(* Logix 5000 AddOnInstructionDefinition export AMCI_3204_AOP_Reset_Errors; software revision 20.03 *)

ADD_ON_INSTRUCTION AMCI_3204_AOP_Reset_Errors   (* revision 1.0, vendor AMCI, ExecuteEnableInFalse *)
VAR_INPUT
   axis_status_bits : INT; {required}
   channel_number : INT; {required}
END_VAR
VAR_IN_OUT
   AMCI_3204_output_data : AM:1756_3204:O:0; {required}
END_VAR
VAR_OUTPUT
   EN : BOOL; {access Read Only, visible}
END_VAR
VAR
   command_data_block : DINT[8]; {access None}
END_VAR

ROUTINE EnableInFalse   (* ladder *)
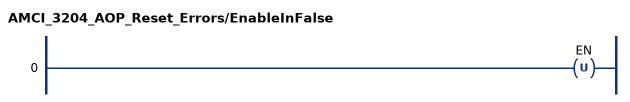
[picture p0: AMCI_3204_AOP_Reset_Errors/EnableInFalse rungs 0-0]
   0: OTU(EN);
END_ROUTINE

ROUTINE Logic   (* ladder *)
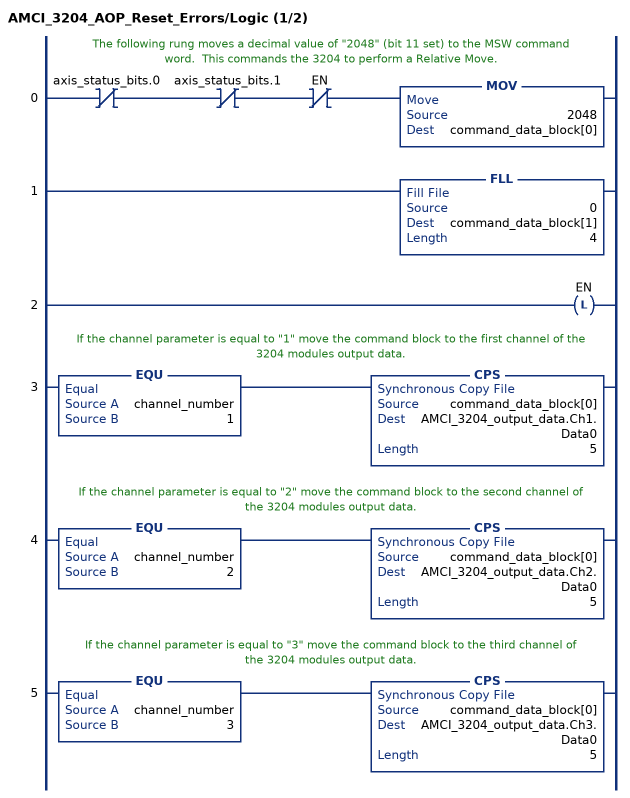
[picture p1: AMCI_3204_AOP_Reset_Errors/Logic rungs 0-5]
   // The following rung moves a decimal value of "2048" (bit 11 set) to the MSW command word.  This commands the 3204 to perform a Relative Move.
   0: XIO(axis_status_bits.0)XIO(axis_status_bits.1)XIO(EN)MOV(2048,command_data_block[0]);
   1: FLL(0,command_data_block[1],4);
   2: OTL(EN);
   // If the channel parameter is equal to "1" move the command block to the first channel of the 3204 modules output data.
   3: EQU(channel_number,1)CPS(command_data_block[0],AMCI_3204_output_data.Ch1.Data0,5);
   // If the channel parameter is equal to "2" move the command block to the second channel of the 3204 modules output data.
   4: EQU(channel_number,2)CPS(command_data_block[0],AMCI_3204_output_data.Ch2.Data0,5);
   // If the channel parameter is equal to "3" move the command block to the third channel of the 3204 modules output data.
   5: EQU(channel_number,3)CPS(command_data_block[0],AMCI_3204_output_data.Ch3.Data0,5);
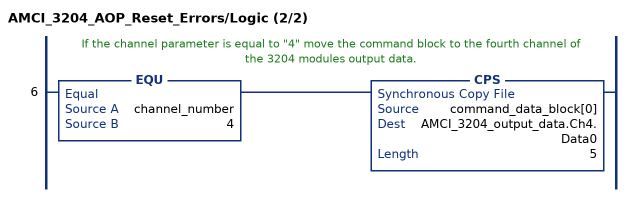
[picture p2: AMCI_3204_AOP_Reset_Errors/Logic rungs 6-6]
   // If the channel parameter is equal to "4" move the command block to the fourth channel of the 3204 modules output data.
   6: EQU(channel_number,4)CPS(command_data_block[0],AMCI_3204_output_data.Ch4.Data0,5);
END_ROUTINE
END_ADD_ON_INSTRUCTION
